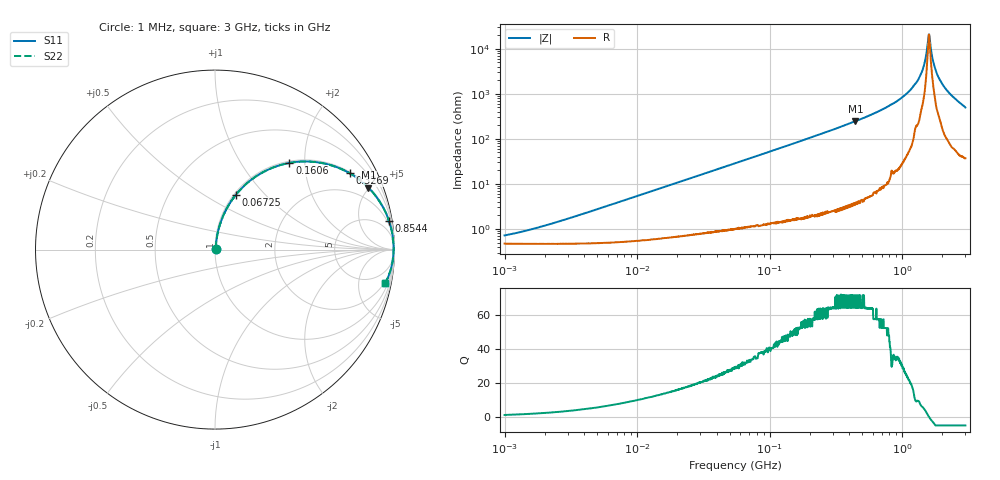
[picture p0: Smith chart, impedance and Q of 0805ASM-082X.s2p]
!s-Parameter Generated by FASTRON Sdn. Bhd.
!FASTRON P/N : 0805ASM-082X
!Keysight Technologies: E4991B_MY54100416_A.01.15
!Date: Fri Jun 19 14:49:52 2026
!Version  :Rev00  Fri Jun 19 14:49:52 2026
!Data & Calibration Information:
!Freq  S11  S21  S12  S22
!PortZ  Port1:50+j0  Port2:50+j0
!When reading reference impedance value at option line is always used.
! Remarks : This data is being provided solely for informational purposes.
# Hz S dB R 50
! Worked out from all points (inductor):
!   1601 points, 1 MHz to 3 GHz, reference 50 ohm
!   read as one part in series: L = 86.3 nH near 2.588 MHz
!   highest Q = 71.3 at 443.6 MHz (marker M1), where L = 88.4 nH
!   self-resonance near 1.589 GHz
!   S11 on the Smith chart (normalised r, x): 1 MHz: 1.01, +0.01; 67.25 MHz: 1.02, +0.70; 160.6 MHz: 1.04, +1.68; 326.9 MHz: 1.05, +3.50; 854.4 MHz: 1, +12; 3 GHz: 2, -10
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1000000  -42.90 48.7  -0.04 -0.3  -0.04 -0.3  -42.90 48.7
3804036  -33.50 75.8  -0.04 -1.2  -0.04 -1.2  -33.50 75.8
1.447069e7  -22.30 81.1  -0.08 -4.4  -0.08 -4.4  -22.30 81.1
5.504702e7  -11.20 72.1  -0.43 -15.9  -0.43 -15.9  -11.20 72.1
6.724529e7  -9.67 69.0  -0.59 -19.2  -0.59 -19.2  -9.67 69.0
1.606197e8  -3.93 49.3  -2.40 -39.5  -2.40 -39.5  -3.93 49.3
2.083556e8  -2.72 42.0  -3.49 -47.0  -3.49 -47.0  -2.72 42.0
3.268837e8  -1.28 29.5  -6.16 -59.7  -6.16 -59.7  -1.28 29.5
4.435663e8  -0.71 22.0  -8.54 -67.2  -8.54 -67.2  -0.71 22.0
7.925923e8  -0.18 10.5  -14.80 -78.3  -14.80 -78.3  -0.18 10.5
8.543737e8  -0.16 9.3  -15.80 -79.1  -15.80 -79.1  -0.16 9.3
1.097256e9  -0.07 5.4  -20.50 -82.1  -20.50 -82.1  -0.07 5.4
1.307284e9  -0.06 2.9  -25.90 -81.1  -25.90 -81.1  -0.06 2.9
1.437675e9  -0.05 1.5  -31.30 -78.1  -31.30 -78.1  -0.05 1.5
1.488926e9  -0.04 1.0  -34.70 -74.5  -34.70 -74.5  -0.04 1.0
1.54974e9  -0.04 0.4  -41.20 -57.8  -41.20 -57.8  -0.04 0.4
1.596974e9  -0.04 -0.0  -46.40 5.0  -46.40 5.0  -0.04 -0.0
1.637435e9  -0.04 -0.4  -41.30 53.2  -41.30 53.2  -0.04 -0.4
1.76507e9  -0.05 -1.5  -31.70 76.2  -31.70 76.2  -0.05 -1.5
1.941122e9  -0.07 -2.9  -25.90 80.0  -25.90 80.0  -0.07 -2.9
2.312676e9  -0.11 -5.8  -19.90 80.0  -19.90 80.0  -0.11 -5.8
3e9  -0.29 -11.1  -14.20 74.6  -14.20 74.6  -0.29 -11.1
